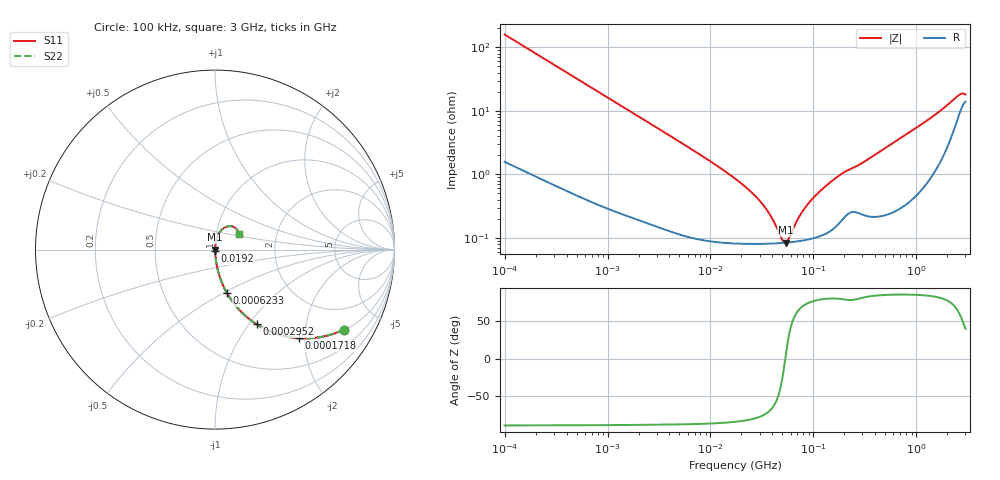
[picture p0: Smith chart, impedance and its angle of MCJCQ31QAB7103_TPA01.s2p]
! MCJCQ31QAB7103_TPA01  S-PARAMETER MODEL  ( Standard Model )
! Model Generated by TAIYO YUDEN Corporation (http://www.ty-top.com)
! Version 1.0
! TAIYO YUDEN Control No. 220601
! Copyright(c) 2015 TAIYO YUDEN CO.,LTD. All Rights Reserved.
! Product Description (link to TY-COMPAS)
! https://ds.yuden.co.jp/TYCOMPAS/or/detail?pn=MCJCQ31QAB7103KTPA01&u=M
! Products Name : Multilayer Ceramic Capacitors
! Characteristics :
!  Capacitance : 0.01 [uF] , Rated Voltage : 250 [V] , TCC : X7R
!  Case Size : 3.2 x 1.6 / 0.126 x 0.063 [mm/inch] , Thickness : 1.15 / 0.045 [mm/inch]
!  (Conditions: Temperature = 25 [degC] , DC Bias Voltage = 0 [V])
! External Node Assignments :
!  1  o---| |---o  2
! GND o---------o GND
! Frequency Range : 100kHz  -  3GHz  [ 401 STEP ]
# MHZ S RI R 50
! Freq[MHz].  S11 Real  S11 Imag  S21 Real  S21 Imag  S12 Real  S12 Imag  S22 Real  S22 Imag
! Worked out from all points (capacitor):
!   401 points, 100 kHz to 3 GHz, reference 50 ohm
!   read as one part in series: C = 9.96 nF near 105.3 kHz
!   lowest |Z| = 84.2 mohm at 53.83 MHz (marker M1)
!   series resonance near 53.35 MHz, so ESL is about 890 pH
!   S11 on the Smith chart (normalised r, x): 100 kHz: 1.03, -3.19; 171.8 kHz: 1.02, -1.86; 295.2 kHz: 1.01, -1.09; 623.3 kHz: 1.01, -0.52; 19.2 MHz: 1.00, -0.02; 3 GHz: 1.28, +0.23
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0.1  0.7162 -0.4459  0.2838 0.4459  0.2838 0.4459  0.7162 -0.4459
0.17181  0.4653 -0.4933  0.5347 0.4933  0.5347 0.4933  0.4653 -0.4933
0.295187  0.2316 -0.4156  0.7684 0.4156  0.7684 0.4156  0.2316 -0.4156
0.562235  0.0796 -0.2633  0.9204 0.2633  0.9204 0.2633  0.0796 -0.2633
0.623288  0.0663 -0.2412  0.9337 0.2412  0.9337 0.2412  0.0663 -0.2412
1.316074  0.0174 -0.1211  0.9826 0.1211  0.9826 0.1211  0.0174 -0.1211
3.161081  0.00412 -0.0515  0.9959 0.0515  0.9959 0.0515  0.00412 -0.0515
17.7727  0.000881 -0.00828  0.9991 0.00828  0.9991 0.00828  0.000881 -0.00828
19.20135  0.000865 -0.0075  0.9991 0.0075  0.9991 0.0075  0.000865 -0.0075
26.16047  0.000825 -0.00481  0.9992 0.00481  0.9992 0.00481  0.000825 -0.00481
32.98988  0.000815 -0.0031  0.9992 0.0031  0.9992 0.0031  0.000815 -0.0031
39.51212  0.000817 -0.00189  0.9992 0.00189  0.9992 0.00189  0.000817 -0.00189
49.82709  0.000831 -0.000424  0.9992 0.000424  0.9992 0.000424  0.000831 -0.000424
53.83243  0.000839 5.63e-05  0.9992 -5.63e-05  0.9992 -5.63e-05  0.000839 5.63e-05
58.15973  0.000849 0.000536  0.9992 -0.000536  0.9992 -0.000536  0.000849 0.000536
75.25761  0.000901 0.00217  0.9991 -0.00217  0.9991 -0.00217  0.000901 0.00217
97.38194  0.00099 0.00396  0.999 -0.00396  0.999 -0.00396  0.00099 0.00396
180.7614  0.00183 0.00958  0.9982 -0.00958  0.9982 -0.00958  0.00183 0.00958
547.5153  0.00318 0.0283  0.9968 -0.0283  0.9968 -0.0283  0.00318 0.0283
1575.075  0.0198 0.0869  0.9802 -0.0869  0.9802 -0.0869  0.0198 0.0869
2441.062  0.0783 0.1307  0.9217 -0.1307  0.9217 -0.1307  0.0783 0.1307
3000  0.1311 0.0886  0.8689 -0.0886  0.8689 -0.0886  0.1311 0.0886
